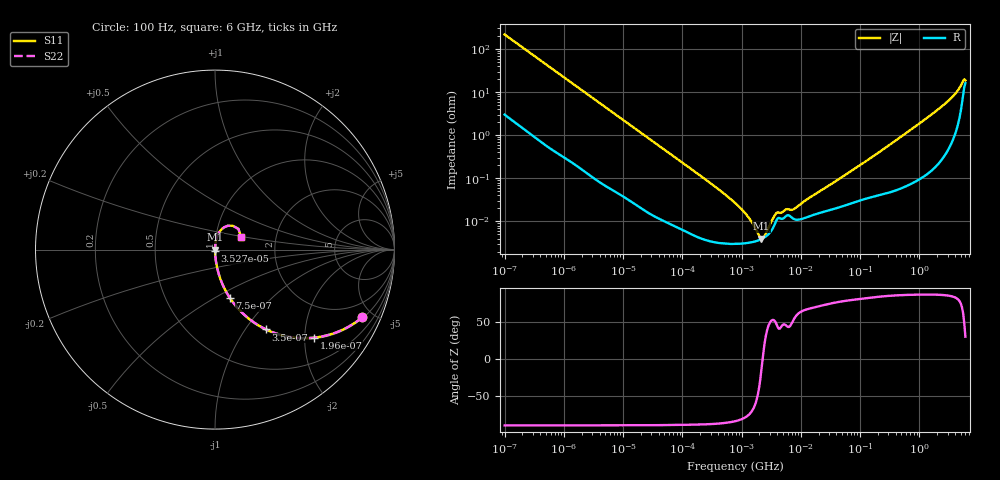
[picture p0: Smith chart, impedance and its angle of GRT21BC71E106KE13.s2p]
!Murata Part Number: GRT21BC71E106KE13
!These Parameters are Measured in Series Mode Connection
!Data Generated on Jun 19, 2026
!  o--ll--o
!Port1  Port2
!  o------o
!Operation Temp=25[degC], DC Bias Voltage=0[V]
!Freq. Start=100[Hz] Stop=6[GHz] 401[Steps]
# Hz S RI R 50
!Freq.(Hz) S11(Real) S11(Imag) S21(Real) S21(Imag) S12(Real) S12(Imag) S22(Real) S22(Imag)
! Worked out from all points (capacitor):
!   401 points, 100 Hz to 6 GHz, reference 50 ohm
!   read as one part in series: C = 7.3 uF near 109 Hz
!   lowest |Z| = 4.02 mohm at 2.169 MHz (marker M1)
!   series resonance near 2.266 MHz, so ESL is about 680 pH
!   S11 on the Smith chart (normalised r, x): 100 Hz: 1.06, -4.34; 196 Hz: 1.03, -2.23; 350 Hz: 1.02, -1.25; 750 Hz: 1.01, -0.59; 35.27 kHz: 1.00, -0.01; 6 GHz: 1.32, +0.19
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100  0.8217 -0.3759  0.1783 0.3759  0.1783 0.3759  0.8217 -0.3759
196  0.554 -0.4904  0.446 0.4904  0.446 0.4904  0.554 -0.4904
350  0.2845 -0.4447  0.7155 0.4447  0.7155 0.4447  0.2845 -0.4447
750  0.0828 -0.269  0.9172 0.269  0.9172 0.269  0.0828 -0.269
2008  0.0137 -0.1092  0.9863 0.1092  0.9863 0.1092  0.0137 -0.1092
6151  0.0019 -0.0365  0.9981 0.0365  0.9981 0.0365  0.0019 -0.0365
35265  0.000169 -0.00649  0.9998 0.00649  0.9998 0.00649  0.000169 -0.00649
40335  0.000148 -0.00568  0.9999 0.00568  0.9999 0.00568  0.000148 -0.00568
302498  3.48e-05 -0.00076  1 0.00076  1 0.00076  3.48e-05 -0.00076
774597  3.02e-05 -0.000268  1 0.000268  1 0.000268  3.02e-05 -0.000268
1449809  3.27e-05 -9.68e-05  1 9.68e-05  1 9.68e-05  3.27e-05 -9.68e-05
2169299  3.91e-05 -9.3e-06  1 9.3e-06  1 9.3e-06  3.91e-05 -9.3e-06
2967816  5.38e-05 6.1e-05  0.9999 -6.1e-05  0.9999 -6.1e-05  5.38e-05 6.1e-05
3882480  0.000106 0.000115  0.9999 -0.000115  0.9999 -0.000115  0.000106 0.000115
5809218  0.000138 0.000135  0.9999 -0.000135  0.9999 -0.000135  0.000138 0.000135
7599586  0.000114 0.000155  0.9999 -0.000155  0.9999 -0.000155  0.000114 0.000155
1.555665e7  0.000139 0.000364  0.9999 -0.000364  0.9999 -0.000364  0.000139 0.000364
3.124326e8  0.000503 0.00591  0.9995 -0.00591  0.9995 -0.00591  0.000503 0.00591
2.450438e9  0.00506 0.0472  0.9949 -0.0472  0.9949 -0.0472  0.00506 0.0472
4.385646e9  0.0256 0.0999  0.9744 -0.0999  0.9744 -0.0999  0.0256 0.0999
5.245841e9  0.0699 0.1324  0.9301 -0.1324  0.9301 -0.1324  0.0699 0.1324
6e9  0.1445 0.0697  0.8555 -0.0697  0.8555 -0.0697  0.1445 0.0697
